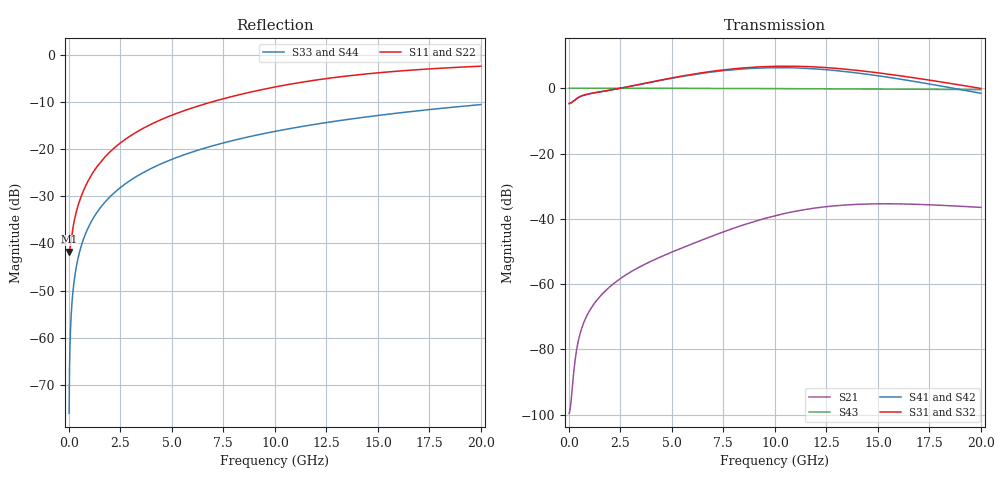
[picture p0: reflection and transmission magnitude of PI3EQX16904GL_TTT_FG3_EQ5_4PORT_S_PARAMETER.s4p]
! NPort=4 DATA=2000 NOISE=0 GROUPDELAY=0 COMPLEX_DATAFORMAT=POLAR
! NumOfBlock=1 NumOfParam=0
! .MODEL Smodel S TSTONEFILE=PI3EQX16904GL_TTT_FG3_EQ5_4PORT_S_PARAMETER.s4p TYPE=S
!  -- The above .MODEL line can be used for the S element in the netlist.
! The s parameter is extracted from the linear redriver, it is not bi-directional; only s(4,1)s(4,2) and s(3,1)s(3,2)
! should be the insertion loss
!Port definition:
!Port1 = input+
!Port2 = input-
!Port3 = output+
!Port4 = output-
# Hz S MA R  50
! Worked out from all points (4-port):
!   2000 points, 10 MHz to 20 GHz, reference 50 ohm
!   strongest paths, dB at 10 MHz, 5.01 GHz, 10.01 GHz, 15.01 GHz, 20 GHz:
!     S31: -4.7, 3.2, 6.7, 4.7, -0.1
!     S32: -4.7, 3.0, 6.6, 4.6, -0.2
!     S41: -4.7, 3.1, 6.3, 3.8, -1.6
!     S42: -4.7, 2.9, 6.2, 3.7, -1.7
!     S43: 0.0, 0.0, -0.1, -0.3, -0.4
!     S21: -99.6, -50.2, -39.1, -35.4, -36.5
!   lowest |S11| = -41.7 dB at 10 MHz (marker M1), VSWR 1.02, Z = 49.2 - j0.0603 ohm
!   |S11| at or under -10 dB: start of sweep to 6.887 GHz
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1e7  0.008182 -175.7  1.05e-05 7.7  0 0.0  0 0.0
     1.05e-05 7.7  0.008182 -175.7  0 0.0  0 0.0
     0.5835 0.5  0.5835 -179.5  0.0001571 -90.0  1 -0.0
     0.5835 -179.6  0.5835 0.4  1 -0.0  0.0001571 -90.0
3.8e8  0.02256 -119.7  0.0001012 117.9  0 0.0  0 0.0
       0.0001012 117.9  0.02256 -119.7  0 0.0  0 0.0
       0.6968 10.1  0.6964 -170.0  0.005969 -90.4  1 -0.3
       0.6968 -170.6  0.6963 9.3  1 -0.3  0.005969 -90.4
1.6e9  0.07608 -102.8  0.0006951 107.4  0 0.0  0 0.0
       0.0006949 107.4  0.07609 -102.8  0 0.0  0 0.0
       0.891 3.0  0.8893 -177.3  0.02512 -91.5  0.9997 -1.4
       0.8899 -179.8  0.8882 -0.2  0.9997 -1.4  0.02512 -91.5
6.02e9  0.2766 -105.0  0.004209 94.4  0 0.0  0 0.0
        0.004177 94.6  0.2766 -105.0  0 0.0  0 0.0
        1.641 -38.9  1.607 140.8  0.09411 -95.6  0.9952 -5.4
        1.611 130.4  1.578 -49.9  0.9952 -5.4  0.09411 -95.6
9.67e9  0.4441 -112.0  0.01055 67.2  0 0.0  0 0.0
        0.01047 68.1  0.4438 -112.0  0 0.0  0 0.0
        2.154 -98.7  2.119 81.5  0.15 -99.0  0.9878 -8.6
        2.057 64.4  2.024 -115.4  0.9878 -8.6  0.15 -99.0
1.359e10  0.6038 -122.0  0.01646 20.9  0 0.0  0 0.0
          0.01639 22.0  0.6034 -122.0  0 0.0  0 0.0
          1.934 -167.7  1.91 12.4  0.2084 -102.5  0.9763 -12.0
          1.773 -10.8  1.752 169.4  0.9763 -12.0  0.2084 -102.5
2e10  0.7639 -136.1  0.01501 -35.5  0 0.0  0 0.0
      0.01497 -33.8  0.7637 -136.0  0 0.0  0 0.0
      0.9923 100.0  0.9814 -80.0  0.2986 -108.1  0.9506 -17.4
      0.8355 -111.9  0.8263 68.1  0.9506 -17.4  0.2986 -108.1
